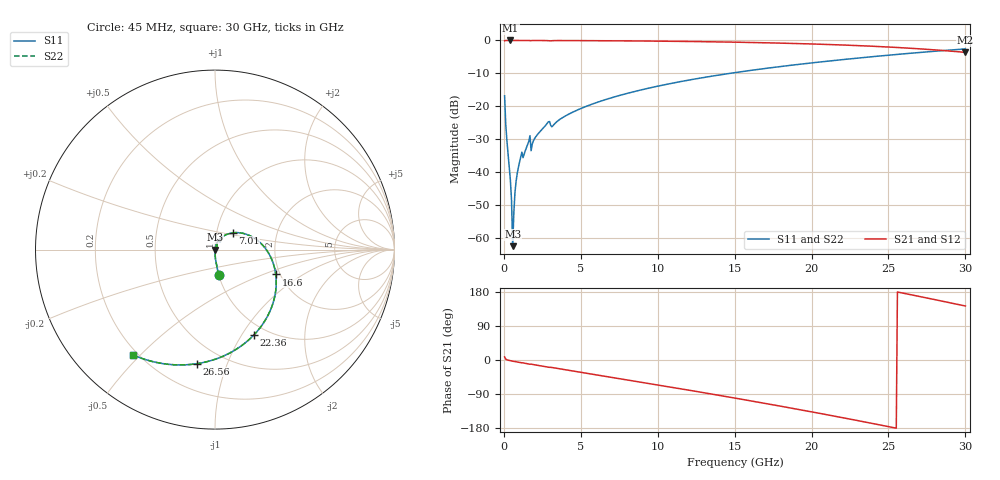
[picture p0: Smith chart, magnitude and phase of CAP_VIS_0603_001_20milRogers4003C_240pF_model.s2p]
! S-parameter model data by Modelithics Inc.  support@modelithics.com  813-866-6335  Tampa FL USA
! S-Parameter data specifications:
! Substrate: 20-mil Rogers 4003C, substrate thickness, H=0.508mm, Dielectric constant, Er=3.75
! PCB Mounting Pad Footprint: Pad width, PadW=0.90mm , Pad length, PadL=1.00mm , Pad gap, PadG (edge-to-edge)=1.00mm , Reference planes=3.0mm apart
! Created Wed Nov 18 13:33:21 2015
# hz S ma R 50
! 2 Port Network Data from SP1.SP block
! freq  magS11  angS11  magS21  angS21  magS12  angS12  magS22  angS22
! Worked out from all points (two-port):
!   401 points, 45 MHz to 30 GHz, reference 50 ohm
!   highest |S21| = 0.00 dB at 419.4 MHz (marker M1); lowest = -3.6 dB at 30 GHz (marker M2)
!   |S21| within 3 dB of the highest: start of sweep to 28.42 GHz
!   lowest |S11| = -62.4 dB at 569.2 MHz (marker M3), VSWR 1.00, Z = 50.1 - j0.0548 ohm
!   |S11| at or under -10 dB: start of sweep to 14.67 GHz
!   |S22| runs from -62.4 to -2.6 dB; largest |S21 - S12| = 0
!   S11 on the Smith chart (normalised r, x): 45 MHz: 1.00, -0.29; 7.01 GHz: 1.19, +0.23; 16.6 GHz: 1.90, -0.61; 22.36 GHz: 0.87, -1.13; 26.56 GHz: 0.36, -0.79; 30 GHz: 0.18, -0.48
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4.5e7  0.1446 -81.8  0.9893 8.1  0.9893 8.1  0.1446 -81.8
1.94775e8  0.03019 -88.7  0.9992 0.7  0.9992 0.7  0.03019 -88.7
3.4455e8  0.01253 -89.1  0.9995 -1.2  0.9995 -1.2  0.01253 -89.1
4.194375e8  0.007641 -88.2  0.9995 -1.8  0.9995 -1.8  0.007641 -88.2
5.692125e8  0.0007578 -46.2  0.9994 -3.1  0.9994 -3.1  0.0007578 -46.2
7.189875e8  0.004963 78.6  0.9993 -4.2  0.9993 -4.2  0.004963 78.6
8.687625e8  0.009695 80.5  0.9992 -5.3  0.9992 -5.3  0.009695 80.5
1.018538e9  0.01437 79.9  0.9989 -6.3  0.9989 -6.3  0.01437 79.9
1.54275e9  0.02624 77.3  0.9982 -9.9  0.9982 -9.9  0.02624 77.3
1.917188e9  0.03005 75.2  0.998 -12.1  0.998 -12.1  0.03005 75.2
2.815838e9  0.05536 67.5  0.9943 -18.4  0.9943 -18.4  0.05536 67.5
3.190275e9  0.05098 64.0  0.9933 -20.2  0.9933 -20.2  0.05098 64.0
5.062462e9  0.09405 56.2  0.9935 -32.8  0.9935 -32.8  0.09405 56.2
7.009538e9  0.1354 43.6  0.9883 -45.7  0.9883 -45.7  0.1354 43.6
1.007992e10  0.2044 23.1  0.9758 -66.3  0.9758 -66.3  0.2044 23.1
1.50225e10  0.3252 -11.0  0.9415 -100.5  0.9415 -100.5  0.3252 -11.0
1.659514e10  0.3656 -22.2  0.9263 -111.8  0.9263 -111.8  0.3656 -22.2
2.003996e10  0.4574 -47.5  0.8839 -137.1  0.8839 -137.1  0.4574 -47.5
2.236148e10  0.5217 -65.3  0.847 -154.9  0.847 -154.9  0.5217 -65.3
2.505742e10  0.5992 -86.6  0.7936 -176.3  0.7936 -176.3  0.5992 -86.6
2.655518e10  0.6431 -98.9  0.7581 171.5  0.7581 171.5  0.6431 -98.9
3e10  0.7438 -127.9  0.659 142.5  0.659 142.5  0.7438 -127.9
